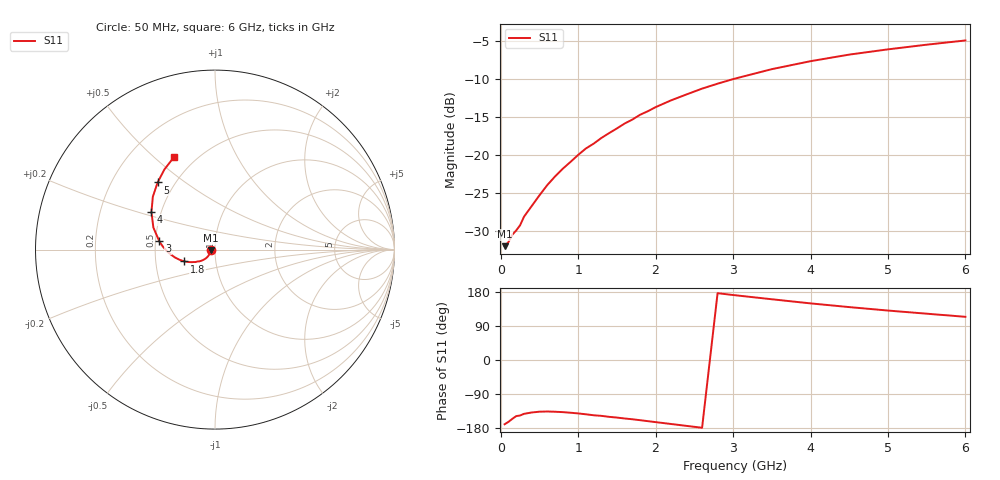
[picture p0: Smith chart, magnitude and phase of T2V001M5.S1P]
! SIEMENS Discrete & RF Semiconductors
! BAS70-04W
! Si Schottky Diode in SOT323
! IF = 1.5 mA
! S-Parameters:  November  1997
# GHz  S  MA  R  50
!  f  S11
! GHz  MAG  ANG
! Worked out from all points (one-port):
!   34 points, 50 MHz to 6 GHz, reference 50 ohm
!   lowest |S11| = -32.0 dB at 50 MHz (marker M1), VSWR 1.05, Z = 47.6 - j0.43 ohm
!   |S11| at or under -10 dB: start of sweep to 3.027 GHz
!   S11 on the Smith chart (normalised r, x): 50 MHz: 0.95, -0.01; 1.8 GHz: 0.70, -0.10; 3 GHz: 0.52, +0.05; 4 GHz: 0.44, +0.22; 5 GHz: 0.40, +0.40; 6 GHz: 0.38, +0.58
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0.05  0.02498 -169.6
0.1  0.02658 -163.2
0.15  0.02971 -155.2
0.2  0.0317 -148.0
0.25  0.03428 -146.4
0.3  0.039 -142.1
0.5  0.05397 -136.4
0.6  0.06292 -135.9
0.7  0.0717 -136.5
0.8  0.08065 -137.6
1  0.09954 -141.0
1.1  0.1098 -143.3
1.2  0.118 -145.8
1.3  0.1287 -147.4
1.6  0.1601 -154.3
1.7  0.17 -156.4
1.8  0.1829 -158.8
2  0.2052 -163.9
2.2  0.2274 -168.9
2.4  0.2488 -173.9
2.6  0.2716 -178.8
3  0.3137 171.5
3.5  0.3647 160.3
4  0.4115 149.4
4.5  0.4547 139.6
5  0.4923 130.5
5.5  0.5284 122.2
6  0.5633 114.0
